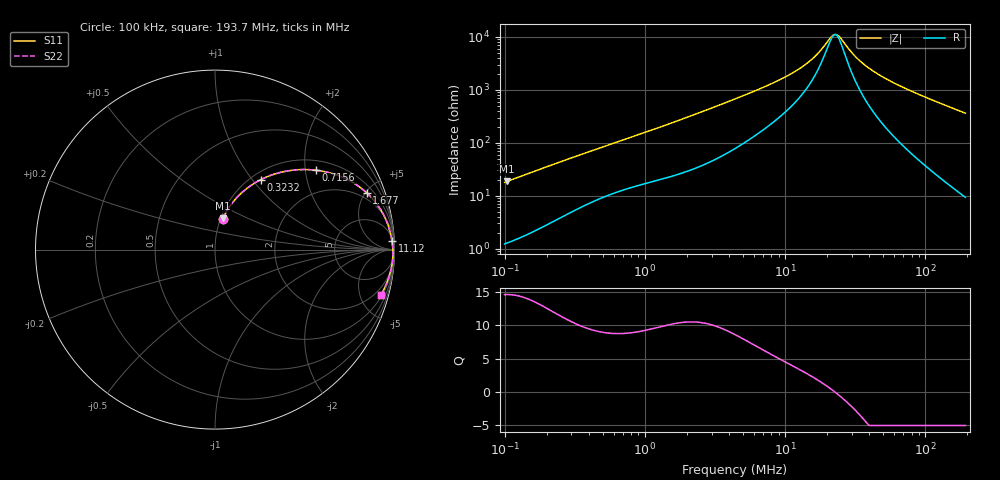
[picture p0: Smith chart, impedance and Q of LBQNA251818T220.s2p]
! LBQNA251818T220  S-PARAMETER MODEL  ( General Type )
! Model Generated by TAIYO YUDEN Corporation (http://www.ty-top.com)
! Version 1.0
! TAIYO YUDEN Control No. 191025NI43SB-FBB
! Copyright(c) 2019 TAIYO YUDEN CO.,LTD. All Rights Reserved.
! Product Description (link to TY-COMPAS)
! https://ds.yuden.co.jp/TYCOMPAS/or/detail?pn=LBQNA251818T220K&u=M
! Products Name : Inductors
! Characteristics :
!  Inductance : 22 uH , SRF(min) : 19 MHz , DC Resistance(max) : 0.65 Ohm
!  Rated Current : Saturation :165 mA , Temp Rise : 390 mA (20 degC)
!  Case Size : 2.5 x 1.8 / 0.098 x 0.071 [mm/inch] , Thickness : 1.8 / 0.071 [mm/inch]
!  (Conditions: Temperature = 25 degC , DC Bias Current/Voltage = 0A / 0V)
! External Node Assignments :
!  1  o---GGG---o  2
! GND o---------o GND
! Frequency Range : 0.1MHz  -  193.730505MHz  [ 402 STEP ]
# MHz S RI R 50
! Freq[MHz].  S11 Real  S11 Imag  S21 Real  S21 Imag  S12 Real  S12 Imag  S22 Real  S22 Imag
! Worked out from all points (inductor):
!   401 points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, 100 kHz to 193.7 MHz, reference 50 ohm
!   read as one part in series: L = 28.3 uH near 103.9 kHz
!   highest Q = 14.6 at 103.9 kHz (marker M1), where L = 28.4 uH
!   self-resonance near 22.41 MHz
!   S11 on the Smith chart (normalised r, x): 100 kHz: 1.02, +0.36; 323.2 kHz: 1.11, +1.11; 715.6 kHz: 1.26, +2.28; 1.677 MHz: 1.49, +5.08; 11.12 MHz: 11, +39; 193.7 MHz: 1.19, -7.24
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0.1  0.0419 0.1691  0.9581 -0.1691  0.9581 -0.1691  0.0419 0.1691
0.103857  0.0446 0.1749  0.9554 -0.1749  0.9554 -0.1749  0.0446 0.1749
0.190288  0.1193 0.2874  0.8807 -0.2874  0.8807 -0.2874  0.1193 0.2874
0.323233  0.2562 0.3902  0.7438 -0.3902  0.7438 -0.3902  0.2562 0.3902
0.355309  0.2882 0.4049  0.7118 -0.4049  0.7118 -0.4049  0.2882 0.4049
0.715602  0.5618 0.4424  0.4382 -0.4424  0.4382 -0.4424  0.5618 0.4424
1.262442  0.7682 0.3737  0.2318 -0.3737  0.2318 -0.3737  0.7682 0.3737
1.6768  0.8441 0.3174  0.1559 -0.3174  0.1559 -0.3174  0.8441 0.3174
2.591165  0.9194 0.2282  0.0806 -0.2282  0.0806 -0.2282  0.9194 0.2282
4.401483  0.9628 0.1399  0.0372 -0.1399  0.0372 -0.1399  0.9628 0.1399
7.619402  0.9804 0.0774  0.0196 -0.0774  0.0196 -0.0774  0.9804 0.0774
11.12451  0.986 0.0465  0.014 -0.0465  0.014 -0.0465  0.986 0.0465
15.63884  0.9891 0.0235  0.0109 -0.0235  0.0109 -0.0235  0.9891 0.0235
21.573  0.9909 0.00329  0.0091 -0.00329  0.0091 -0.00329  0.9909 0.00329
23.26926  0.9912 -0.00144  0.00884 0.00144  0.00884 0.00144  0.9912 -0.00144
24.62842  0.9913 -0.00501  0.00868 0.00501  0.00868 0.00501  0.9913 -0.00501
30.32735  0.9916 -0.0185  0.00844 0.0185  0.00844 0.0185  0.9916 -0.0185
35.28405  0.9914 -0.0289  0.00861 0.0289  0.00861 0.0289  0.9914 -0.0289
43.44866  0.9906 -0.0443  0.00941 0.0443  0.00941 0.0443  0.9906 -0.0443
55.56615  0.9886 -0.0652  0.0114 0.0652  0.0114 0.0652  0.9886 -0.0652
96.1905  0.9766 -0.127  0.0234 0.127  0.0234 0.127  0.9766 -0.127
193.7305  0.9236 -0.2531  0.0764 0.2531  0.0764 0.2531  0.9236 -0.2531
